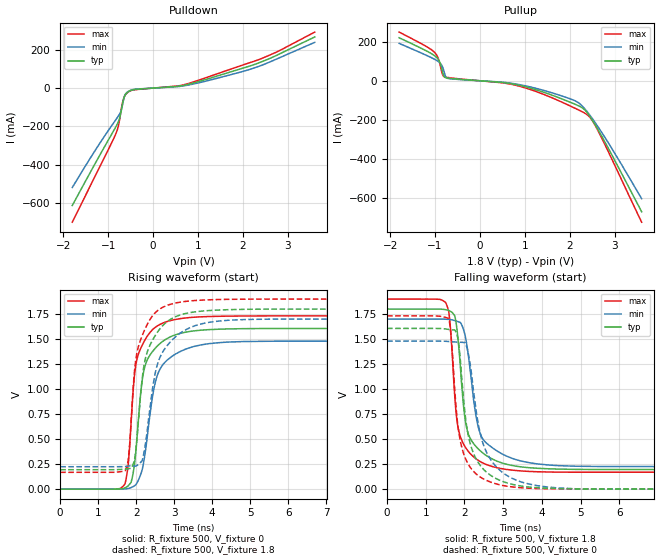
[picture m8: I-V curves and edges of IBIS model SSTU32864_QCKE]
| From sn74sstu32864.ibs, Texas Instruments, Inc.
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[Model]   SSTU32864_QCKE
Model_type  Output
Vref =   1.8
Rref =   1000
Cref =   30p
Vmeas =   0.9
| variable   typ   min   max
C_comp   4.54pF   3.63pF   5.50pF
| C_pullup   4.56pF   3.63pF   5.50pF
| C_pulldown   4.53pF   3.73pF   5.14pF
[Temperature Range]   40   85   0
| Ambient temperature   25   70   0
[Voltage range]   1.8   1.7   1.9
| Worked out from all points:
|   slope of the pulldown table from 0 to 0.27 V, typ, clamps not added: 60.6 ohm
|   slope of the pullup table from 0 to 0.27 V, typ, clamps not added: 59.5 ohm
|   rising waveform, R_fixture 500, V_fixture 0: 20-80 % time 308ps typ, 397ps min, 282ps max; typ from 0 V to 1.61 V
|   falling waveform, R_fixture 500, V_fixture 1.8: 20-80 % time 299ps typ, 370ps min, 254ps max; typ from 1.8 V to 0.195 V
|   rising waveform, R_fixture 500, V_fixture 1.8: 20-80 % time 393ps typ, 488ps min, 339ps max; typ from 0.195 V to 1.8 V
|   falling waveform, R_fixture 500, V_fixture 0: 20-80 % time 379ps typ, 503ps min, 302ps max; typ from 1.61 V to 0 V
[Pulldown]
| SSTU32864_QCKE
|   Voltage   I(typ)   I(min)   I(max)
-1.8V     -613.5mA   -519.3mA   -700.4mA
-840mV    -206.5mA   -168.5mA   -244.1mA
-785mV    -181.7mA   -149.7mA   -207.8mA
-745mV    -156.6mA   -134.7mA   -162.6mA
-705mV    -112.3mA   -111.9mA   -105.3mA
-665mV    -63.66mA   -69.05mA   -61.98mA
-620mV    -34.48mA   -33.38mA   -36.65mA
-560mV    -20.07mA   -18.55mA   -21.69mA
-395mV    -6.837mA   -5.787mA   -8.284mA
880mV     25.3mA     20.45mA    30.74mA
2.26V     123.5mA    106mA      141mA
3.6V      267mA      238.9mA    292.5mA
[Pullup]
| SSTU32864_QCKE
|   Voltage   I(typ)   I(min)   I(max)
-1.8V     219.6mA    190.8mA    248.4mA
-1.015V   128.7mA    110.2mA    145.7mA
-905mV    99.65mA    93.87mA    96.4mA
-840mV    50.49mA    74.02mA    36.2mA
-790mV    19.46mA    38.8mA     19.92mA
-700mV    13.37mA    11.24mA    16.34mA
870mV     -22.69mA   -19.2mA    -27.2mA
2.075V    -115.6mA   -97.82mA   -135.5mA
2.39V     -163.4mA   -158.5mA   -173.5mA
2.505V    -201.9mA   -193.6mA   -204.2mA
2.67V     -265.7mA   -248.8mA   -273.3mA
3.6V      -667.9mA   -601.5mA   -721.3mA
[Ramp]
| SSTU32864_QCKE
| variable   typ   min   max
dV/dt_r   0.96/3.14E-10   0.89/4.09E-10   1.04/2.87E-10
dV/dt_f   0.96/3.02E-10   0.89/3.89E-10   1.04/2.63E-10
R_load = 500
[Rising Waveform]
| SSTU32864_QCKE
R_fixture =   500
C_fixture =   0
L_fixture =   0
V_fixture =   0
V_fixture_min = 0
V_fixture_max = 0
|   Time   V(typ)   V(min)   V(max)
0s        395.3nV    2.664uV    74.81nV
1.705ns   13.9mV     2.818mV    51.87mV
1.8ns     37.1mV     7.778mV    282.4mV
1.915ns   148.6mV    24.92mV    953.7mV
2.075ns   764.2mV    104.2mV    1.366V
2.235ns   1.232V     357.4mV    1.493V
2.42ns    1.37V      899.4mV    1.59V
2.565ns   1.433V     1.146V     1.633V
3.295ns   1.569V     1.398V     1.711V
40ns      1.606V     1.479V     1.732V
[Falling Waveform]
| SSTU32864_QCKE
R_fixture =   500
C_fixture =   0
L_fixture =   0
V_fixture =   1.8
V_fixture_min = 1.7
V_fixture_max = 1.9
|   Time   V(typ)   V(min)   V(max)
0s        1.8V       1.7V       1.9V
1.515ns   1.794V     1.698V     1.866V
1.62ns    1.781V     1.695V     1.689V
1.755ns   1.725V     1.684V     898.7mV
1.895ns   1.22V      1.666V     522.8mV
2.06ns    605.6mV    1.446V     396.7mV
2.265ns   440.2mV    813.4mV    311.8mV
2.4ns     384.7mV    563.8mV    275.6mV
3.225ns   235.3mV    307.3mV    188.6mV
40ns      194.5mV    224.2mV    168.3mV
[Rising Waveform]
| SSTU32864_QCKE
R_fixture =   500
C_fixture =   0
L_fixture =   0
V_fixture =   1.8
V_fixture_min = 1.7
V_fixture_max = 1.9
|   Time   V(typ)   V(min)   V(max)
0s        194.5mV    224.2mV    168.3mV
1.705ns   200.9mV    226.7mV    183.7mV
1.79ns    203.8mV    230.4mV    284.4mV
1.87ns    210.6mV    232.5mV    694.8mV
2.015ns   477.4mV    235.7mV    1.351V
2.165ns   1.124V     294.2mV    1.54V
2.305ns   1.385V     627.1mV    1.656V
2.615ns   1.597V     1.306V     1.798V
3.33ns    1.758V     1.598V     1.878V
40ns      1.8V       1.7V       1.9V
[Falling Waveform]
| SSTU32864_QCKE
R_fixture =   500
C_fixture =   0
L_fixture =   0
V_fixture =   0
V_fixture_min = 0
V_fixture_max = 0
|   Time   V(typ)   V(min)   V(max)
0s        1.606V     1.479V     1.732V
1.595ns   1.596V     1.475V     1.707V
1.835ns   1.499V     1.469V     618.2mV
2.02ns    736.9mV    1.463V     310.6mV
2.185ns   407.8mV    1.143V     198.6mV
2.335ns   277mV      700.2mV    139.8mV
2.485ns   199.6mV    448.2mV    101.6mV
3.235ns   46.35mV    105.7mV    20.41mV
5.64ns    -498.4uV   -2.078mV   -866.5uV
40ns      395.3nV    2.664uV    74.72nV
